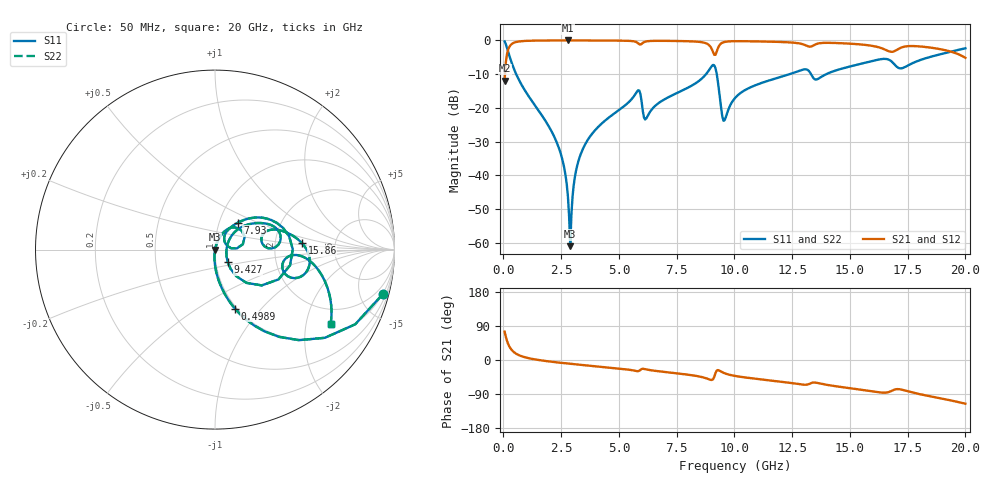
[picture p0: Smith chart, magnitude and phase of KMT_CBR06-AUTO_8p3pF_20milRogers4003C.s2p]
! Data measured by Modelithics Inc. support@modelithics.com 813-866-6335
! KEMET CBR06-AUTO 8.3pF, Pad Width= 0.851mm, Pad Length= 0.64mm, Pad Gap= 0.62mm, 20mil Rogers 4003C substrate Data, January 2022
# hz S ma R 50
! 2 Port Network Data from SP1.SP block
! freq  magS11  angS11  magS21  angS21  magS12  angS12  magS22  angS22
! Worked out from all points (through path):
!   401 points, 50 MHz to 20 GHz, reference 50 ohm
!   highest |S21| = -0.01 dB at 2.793 GHz (marker M1); lowest = -11.9 dB at 50 MHz (marker M2)
!   group delay of S21, straight-line fit = 16.1 ps
!   lowest |S11| = -61.0 dB at 2.893 GHz (marker M3), VSWR 1.00, Z = 50.1 - j0.00322 ohm
!   |S11| at or under -10 dB: 551 MHz to 8.771 GHz (8.22 GHz wide, 176 % of centre); 9.234 GHz to 12.39 GHz (3.157 GHz wide, 29.2 % of centre); 13.32 GHz to 13.98 GHz (659.2 MHz wide, 4.83 % of centre)
!   |S22| runs from -61.0 to -0.3 dB; largest |S21 - S12| = 0
!   S11 on the Smith chart (normalised r, x): 50 MHz: 0.98, -7.53; 498.9 MHz: 0.98, -0.73; 7.93 GHz: 1.22, +0.38; 9.427 GHz: 1.14, -0.16; 15.86 GHz: 2.86, +0.27; 20 GHz: 1.40, -2.78
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5e7  0.9671 -14.9  0.254 75.1  0.254 75.1  0.9671 -14.9
2.495e8  0.6036 -53.7  0.7966 36.3  0.7966 36.3  0.6036 -53.7
4.98875e8  0.3474 -71.3  0.9371 18.6  0.9371 18.6  0.3474 -71.3
2.294375e9  0.03152 -94.6  0.9986 -6.1  0.9986 -6.1  0.03152 -94.6
2.6435e9  0.01224 -94.4  0.999 -8.4  0.999 -8.4  0.01224 -94.4
2.793125e9  0.004776 -88.9  0.999 -9.3  0.999 -9.3  0.004776 -88.9
2.892875e9  0.0008899 -2.1  0.999 -10.0  0.999 -10.0  0.0008899 -2.1
3.14225e9  0.01167 74.0  0.9989 -11.5  0.9989 -11.5  0.01167 74.0
3.391625e9  0.02259 74.6  0.9987 -13.0  0.9987 -13.0  0.02259 74.6
5.785625e9  0.1748 42.9  0.9328 -29.4  0.9328 -29.4  0.1748 42.9
6.184625e9  0.06976 40.0  0.968 -24.8  0.968 -24.8  0.06976 40.0
6.73325e9  0.1189 57.1  0.9863 -29.8  0.9863 -29.8  0.1189 57.1
7.93025e9  0.1947 49.9  0.9744 -38.3  0.9744 -38.3  0.1947 49.9
9.077375e9  0.4333 0.3  0.6679 -50.5  0.6679 -50.5  0.4333 0.3
9.4265e9  0.09874 -44.4  0.9035 -30.7  0.9035 -30.7  0.09874 -44.4
9.576125e9  0.06551 6.8  0.9499 -35.0  0.9499 -35.0  0.06551 6.8
1.0025e10  0.1398 41.5  0.9741 -42.0  0.9741 -42.0  0.1398 41.5
1.336662e10  0.2948 1.6  0.8248 -60.0  0.8248 -60.0  0.2948 1.6
1.586038e10  0.4853 4.3  0.8421 -81.9  0.8421 -81.9  0.4853 4.3
1.670825e10  0.5131 -15.9  0.6873 -84.0  0.6873 -84.0  0.5131 -15.9
1.805488e10  0.5134 -5.7  0.8131 -90.6  0.8131 -90.6  0.5134 -5.7
2e10  0.7651 -32.6  0.5527 -115.2  0.5527 -115.2  0.7651 -32.6
